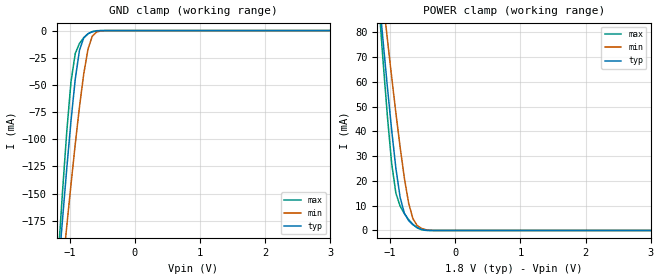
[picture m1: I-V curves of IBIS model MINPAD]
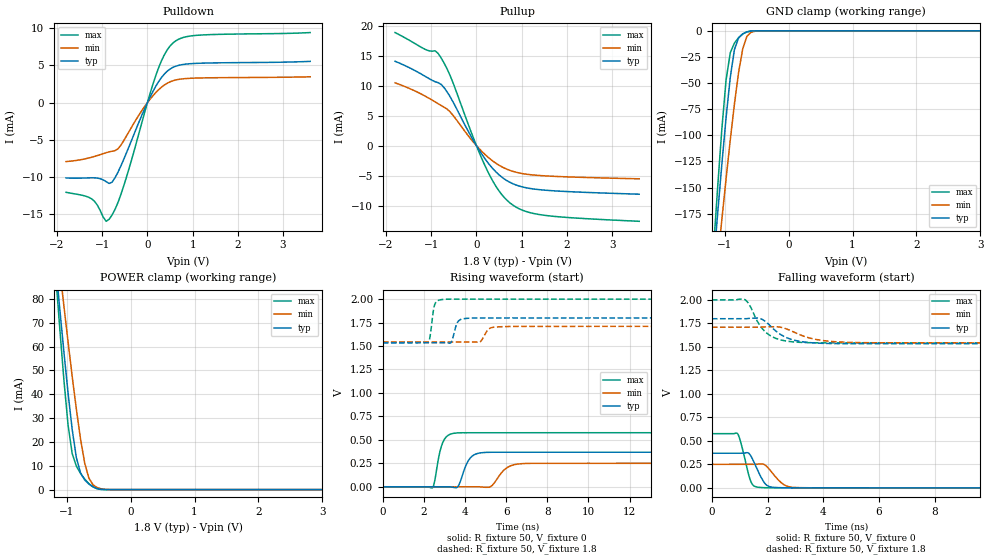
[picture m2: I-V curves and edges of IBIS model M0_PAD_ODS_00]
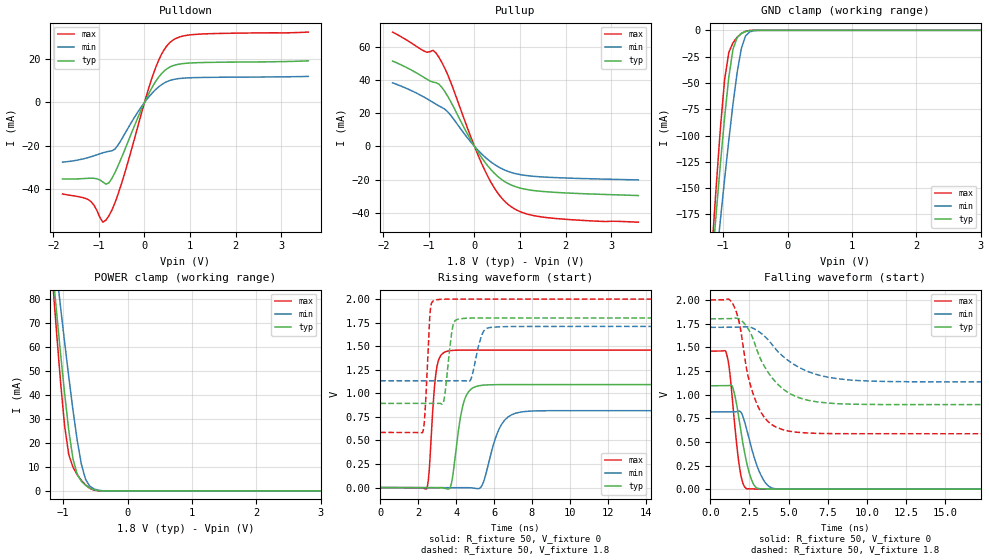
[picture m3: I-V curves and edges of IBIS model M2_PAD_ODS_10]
| Created by SiliconSmart  S-2021.06-SP5-2
[IBIS Ver]   4.0
[File Name]   as320ck_18v_rev1p1.ibs
[File Rev]   1.1
[Date]   Tue Aug 20 2024
|[Source]   Avalanche Team
|[Notes]   Generated IBIS models from Silicon Smart
|[Rev 1.0]   Initial release based on extracted netlist
|[Rev 1.1]   Updated the VCC supply values according to
|		datasheet
|[Disclaimer]   THE MODEL LIBRARIES ARE PROVIDED AS IS.
|[Copyright]   Copyright 2024, Avalanche Technology, All Rights Reserved
[Component]   AS30XX20X_BGA
[Manufacturer]  Avalanche Technology
| CONTENT :
| This file contains IBIS MODEL for PSRAM device
| AS30XX20X
| USAGE :
| The models are derived for the 1.71V to 2.0V I/O Operation.
| Temperatures for model generation: typ: 25, max: -40, min: 125
| Voltages : typ: 1.8V, min: 1.71V, max: 2.0V
| PACKAGES SUPPORTED :
| 56-ball FBGA (10mm x 10mm)
| VERIFICATION
| Errors  : 0
| Warnings: 11
| All warnings due to non-monotonic data:
[Package]
|  Design die-package: BGA
| variable   typ   min   max
R_pkg   0.72029   0.51528   1.0002
L_pkg   5.797e-9   4.155e-9   8.073e-9
C_pkg   1.116e-12   7.907e-13   1.753e-12
|Pin and Model info
[Pin]  signal_name  model_name   R_pin   L_pin   C_pin
E2   CS1#   MINPAD   0.4340	15.2000E-9	1.2600E-12
C3   CS2#   MINPAD   0.3800	13.5000E-9	1.0400E-12
D2   CLK1   MINPAD   0.4300	12.7000E-9	0.9790E-12
D1   CLK2   MINPAD   0.4480	14.6000E-9	1.1600E-12
F3   IO_0   MIOPAD   0.4010	12.4000E-9	1.2500E-12
F2   IO_1   MIOPAD   0.4050	14.2000E-9	1.1100E-12
E4   IO_2   MIOPAD   0.3780	11.8000E-9	1.2000E-12
F4   IO_3   MIOPAD   0.3700	11.8000E-9	1.2600E-12
F5   IO_4   MIOPAD   0.3710	11.1000E-9	1.1000E-12
G3   IO_5   MIOPAD   0.4050	13.8000E-9	1.1600E-12
G2   IO_6   MIOPAD   0.3830	15.2000E-9	1.0900E-12
G1   IO_7   MIOPAD   0.4480	16.4000E-9	1.0800E-12
C7   HTBSEL   MINPAD   0.1380	6.1700E-9	0.6060E-12
B7   HBP_2   MINPAD   0.1470	6.3900E-9	1.0000E-12
A6   HBP_1   MINPAD   0.1910	8.5000E-9	1.1500E-12
A5   HBP_0   MINPAD   0.2050	8.6800E-9	1.4200E-12
C4   RESET#   MINPAD   0.3410	14.1000E-9	1.6300E-12
C5   INT1#   MIOPAD   0.3080	12.5000E-9	1.2100E-12
D3   INT2#   MIOPAD   0.2120	10.3000E-9	0.8230E-12
B1   VSSIO   GND   NA   NA   NA
B5   VSSIO   GND   NA   NA   NA
B6   VSSIO   GND   NA   NA   NA
E1   VSSIO   GND   NA   NA   NA
G5   VSSIO   GND   NA   NA   NA
G6   VSSIO   GND   NA   NA   NA
A1   VSS   GND   NA   NA   NA
A3   VSS   GND   NA   NA   NA
B3   VSS   GND   NA   NA   NA
E5   VSS   GND   NA   NA   NA
E6   VSS   GND   NA   NA   NA
E7   VSS   GND   NA   NA   NA
G7   VSS   GND   NA   NA   NA
A8   VSS   GND   NA   NA   NA
A7   VCCIO   POWER   NA   NA   NA
B2   VCCIO   POWER   NA   NA   NA
B4   VCCIO   POWER   NA   NA   NA
C6   VCCIO   POWER   NA   NA   NA
F1   VCCIO   POWER   NA   NA   NA
F6   VCCIO   POWER   NA   NA   NA
G4   VCCIO   POWER   NA   NA   NA
A2   VCC   POWER   NA   NA   NA
A4   VCC   POWER   NA   NA   NA
D4   VCC   POWER   NA   NA   NA
D6   VCC   POWER   NA   NA   NA
D7   VCC   POWER   NA   NA   NA
F7   VCC   POWER   NA   NA   NA
| IOPAD
[Model Selector] MIOPAD
| Model Description
M0_PAD_ODS_00   35ohms
M1_PAD_ODS_01   40ohms
M2_PAD_ODS_10   20ohms
M3_PAD_ODS_11   15ohms
| Models and submodels in the file (5): MINPAD (Input), M0_PAD_ODS_00 (I/O), M2_PAD_ODS_10 (I/O), M1_PAD_ODS_01 (I/O), M3_PAD_ODS_11 (I/O)
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[Model] MINPAD
Model_type Input
Enable   Active-High
Vinl  =  0.63
Vinh  =  1.17
| Capacitance  typ   min   max
C_comp   1.623824e-12   1.523246e-12   1.739467e-12
| Variables   typ   min   max
[GND Clamp Reference]   0   0   0
[POWER Clamp Reference]   1.8   1.71   2
[Pulldown Reference]   0   0   0
[Pullup Reference]   1.8   1.71   2
[Temperature Range]   25   125   -40
[Voltage Range]   1.8   1.71   2
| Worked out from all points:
|   GND clamp passes 1 mA (typ) near -0.64 V on its own axis
|   POWER clamp passes 1 mA (typ) near -0.57 V on its own axis
[GND Clamp]
| Voltage   I(typ)   I(min)   I(max)
-1.8V     -720.4mA   -670.5mA   -825.2mA
-1.173V   -222.3mA   -260.3mA   -207.5mA
-1.108V   -173.8mA   -219.8mA   -148.3mA
-1.043V   -126.9mA   -180.1mA   -93.11mA
-977.6mV  -83.02mA   -141.5mA   -47mA
-912.4mV  -44.68mA   -104.6mA   -21.04mA
-847.2mV  -17.95mA   -70.1mA    -11.75mA
-782.1mV  -6.736mA   -39.85mA   -6.524mA
-716.9mV  -2.917mA   -17.13mA   -2.959mA
-651.7mV  -1.107mA   -5.246mA   -906.9uA
-456.2mV  -3.885uA   -74.14uA   -372.9nA
3.6V      0A         0A         0A
[POWER Clamp]
| Voltage   I(typ)   I(min)   I(max)
-1.8V     287.1mA    268.3mA    329.6mA
-1.173V   94.89mA    108.5mA    91.02mA
-1.108V   76.1mA     92.66mA    67.97mA
-1.043V   57.9mA     77.16mA    46.14mA
-977.6mV  40.62mA    62.05mA    27.14mA
-912.4mV  25.13mA    47.46mA    15.06mA
-847.2mV  13.38mA    33.64mA    9.853mA
-716.9mV  4.014mA    11.09mA    4.394mA
-651.7mV  2.34mA     4.821mA    2.483mA
-586.6mV  1.18mA     2.003mA    1.113mA
-325.9mV  1.153uA    19.85uA    110.1nA
3.6V      0A         0A         0A
[Model] M0_PAD_ODS_00
Model_type I/O
Enable   Active-High
Vinl  =  0.63
Vinh  =  1.17
Vmeas =  0.9
Cref  =  30e-12
| Capacitance  typ   min   max
C_comp   1.624629e-12   1.520611e-12   1.744819e-12
| Variables   typ   min   max
[GND Clamp Reference]   0   0   0
[POWER Clamp Reference]   1.8   1.71   2
[Pulldown Reference]   0   0   0
[Pullup Reference]   1.8   1.71   2
[Temperature Range]   25   125   -40
[Voltage Range]   1.8   1.71   2
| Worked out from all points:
|   slope of the pulldown table from 0 to 0.27 V, typ, clamps not added: 89.8 ohm
|   slope of the pullup table from 0 to 0.27 V, typ, clamps not added: 90.2 ohm
|   GND clamp passes 1 mA (typ) near -0.64 V on its own axis
|   POWER clamp passes 1 mA (typ) near -0.57 V on its own axis
|   falling waveform, R_fixture 50, V_fixture 0: 20-80 % time 364ps typ, 457ps min, 286ps max; typ from 0.368 V to 0 V
|   falling waveform, R_fixture 50, V_fixture 1.8: 20-80 % time 772ps typ, 993ps min, 609ps max; typ from 1.8 V to 1.53 V
|   rising waveform, R_fixture 50, V_fixture 0: 20-80 % time 416ps typ, 571ps min, 331ps max; typ from 0 V to 0.368 V
|   rising waveform, R_fixture 50, V_fixture 1.8: 20-80 % time 214ps typ, 282ps min, 164ps max; typ from 1.53 V to 1.8 V
[GND Clamp]
| Voltage   I(typ)   I(min)   I(max)
-1.8V     -720.4mA   -670.5mA   -825.2mA
-1.173V   -222.3mA   -260.3mA   -207.5mA
-1.108V   -173.8mA   -219.8mA   -148.3mA
-1.043V   -126.9mA   -180.1mA   -93.11mA
-977.6mV  -83.02mA   -141.5mA   -47.01mA
-912.4mV  -44.68mA   -104.6mA   -21.04mA
-847.2mV  -17.95mA   -70.1mA    -11.75mA
-782.1mV  -6.736mA   -39.85mA   -6.526mA
-716.9mV  -2.917mA   -17.13mA   -2.96mA
-651.7mV  -1.107mA   -5.246mA   -907.6uA
-456.2mV  -3.886uA   -74.14uA   -373.5nA
3.6V      0A         0A         0A
[POWER Clamp]
| Voltage   I(typ)   I(min)   I(max)
-1.8V     287.1mA    268.3mA    329.6mA
-1.173V   94.89mA    108.5mA    91.02mA
-1.108V   76.1mA     92.66mA    67.97mA
-1.043V   57.9mA     77.16mA    46.14mA
-977.6mV  40.62mA    62.05mA    27.14mA
-912.4mV  25.13mA    47.46mA    15.06mA
-847.2mV  13.38mA    33.64mA    9.853mA
-716.9mV  4.014mA    11.09mA    4.394mA
-651.7mV  2.34mA     4.821mA    2.483mA
-586.6mV  1.18mA     2.003mA    1.113mA
-325.9mV  1.153uA    19.85uA    110.1nA
3.6V      0A         0A         0A
[Pulldown]
| Voltage   I(typ)   I(min)   I(max)
-1.8V     -10.11mA   -7.903mA   -12.02mA
-1.238V   -10.08mA   -7.332mA   -12.89mA
-912.4mV  -10.6mA    -6.719mA   -15.91mA
-847.2mV  -10.84mA   -6.607mA   -15.64mA
-716.9mV  -10.08mA   -6.433mA   -14.32mA
-521.4mV  -7.576mA   -5.077mA   -11.12mA
-65.17mV  -872uA     -545.4uA   -1.404mA
248.3mV   2.817mA    1.73mA     4.683mA
434.5mV   4.193mA    2.586mA    7.041mA
620.7mV   4.869mA    3.026mA    8.258mA
1.179V    5.284mA    3.307mA    9.058mA
3.6V      5.531mA    3.462mA    9.391mA
[Pullup]
| Voltage   I(typ)   I(min)   I(max)
-1.8V     14.09mA    10.49mA    18.88mA
-1.108V   11.46mA    8.165mA    15.99mA
-912.4mV  10.68mA    7.305mA    15.83mA
-782.1mV  10.23mA    6.709mA    14.67mA
-586.6mV  8.225mA    5.675mA    11.78mA
-65.17mV  837.2uA    571.9uA    1.256mA
248.3mV   -2.788mA   -1.868mA   -4.273mA
496.6mV   -4.844mA   -3.246mA   -7.521mA
744.8mV   -6.13mA    -4.13mA    -9.572mA
1.055V    -6.951mA   -4.705mA   -10.87mA
1.49V     -7.407mA   -5.024mA   -11.6mA
3.6V      -8.097mA   -5.528mA   -12.62mA
[Ramp]
dV/dt_r   0.221023/0.415541n  0.150294/0.570736n  0.34588/0.331259n
dV/dt_f   0.159898/0.772458n  0.100157/0.992769n  0.274317/0.608956n
R_load = 50
[Falling Waveform]
R_fixture = 50
V_fixture = 0
V_fixture_min = 0
V_fixture_max = 0
| Time   V(typ)   V(min)   V(max)
0s        368.4mV    250.5mV    576.5mV
917.7ps   368.8mV    250.7mV    577.9mV
1.025ns   368.8mV    250.8mV    496.9mV
1.4ns     338.8mV    250.9mV    66.57mV
1.498ns   281.8mV    250.9mV    22.51mV
1.747ns   123.1mV    255.1mV    3.988mV
2.065ns   13.03mV    196.9mV    1.112mV
2.606ns   1.316mV    29.83mV    229.5uV
3.024ns   433.5uV    3.545mV    224.5uV
21.88ns   79.75nV    25.29nV    -226nV
[Falling Waveform]
R_fixture = 50
V_fixture = 1.8
V_fixture_min = 1.71
V_fixture_max = 2
| Time   V(typ)   V(min)   V(max)
0s        1.8V       1.71V      2V
1.175ns   1.8V       1.71V      2.005V
1.306ns   1.803V     1.71V      1.967V
1.72ns    1.803V     1.711V     1.731V
1.981ns   1.756V     1.714V     1.644V
2.418ns   1.642V     1.711V     1.579V
2.948ns   1.572V     1.658V     1.552V
3.916ns   1.539V     1.571V     1.544V
5.337ns   1.534V     1.546V     1.543V
21.88ns   1.534V     1.543V     1.543V
[Rising Waveform]
R_fixture = 50
V_fixture = 0
V_fixture_min = 0
V_fixture_max = 0
| Time   V(typ)   V(min)   V(max)
0s        2.923nV    85.23nV    2.501nV
2.41ns    -265.6uV   -270.7uV   -11.22mV
2.91ns    -320.8uV   -327uV     469.9mV
3.456ns   -7.235mV   -388.3uV   570.2mV
3.683ns   11.84mV    -413.8uV   574.5mV
4.261ns   309.1mV    -478.8uV   575.7mV
4.837ns   363.6mV    -3.076mV   575.7mV
6.059ns   367.9mV    206.6mV    575.8mV
6.73ns    367.9mV    245.7mV    575.8mV
21.88ns   368.4mV    250.5mV    576.5mV
[Rising Waveform]
R_fixture = 50
V_fixture = 1.8
V_fixture_min = 1.71
V_fixture_max = 2
| Time   V(typ)   V(min)   V(max)
0s        1.534V     1.543V     1.543V
2.209ns   1.534V     1.543V     1.54V
2.511ns   1.534V     1.543V     1.934V
2.877ns   1.534V     1.543V     1.996V
3.303ns   1.535V     1.543V     2V
3.663ns   1.763V     1.543V     2V
4.153ns   1.796V     1.542V     2V
4.701ns   1.799V     1.542V     2V
5.68ns    1.799V     1.705V     2V
21.88ns   1.8V       1.71V      2V
[Model] M2_PAD_ODS_10
Model_type I/O
Enable   Active-High
Vinl  =  0.63
Vinh  =  1.17
Vmeas =  0.9
Cref  =  30e-12
| Capacitance  typ   min   max
C_comp   1.624629e-12   1.520611e-12   1.744819e-12
| Variables   typ   min   max
[GND Clamp Reference]   0   0   0
[POWER Clamp Reference]   1.8   1.71   2
[Pulldown Reference]   0   0   0
[Pullup Reference]   1.8   1.71   2
[Temperature Range]   25   125   -40
[Voltage Range]   1.8   1.71   2
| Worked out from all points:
|   slope of the pulldown table from 0 to 0.27 V, typ, clamps not added: 25.7 ohm
|   slope of the pullup table from 0 to 0.27 V, typ, clamps not added: 24.7 ohm
|   GND clamp passes 1 mA (typ) near -0.64 V on its own axis
|   POWER clamp passes 1 mA (typ) near -0.57 V on its own axis
|   falling waveform, R_fixture 50, V_fixture 0: 20-80 % time 706ps typ, 900ps min, 524ps max; typ from 1.09 V to 0 V
|   falling waveform, R_fixture 50, V_fixture 1.8: 20-80 % time 1.87ns typ, 2.55ns min, 1.16ns max; typ from 1.8 V to 0.893 V
|   rising waveform, R_fixture 50, V_fixture 0: 20-80 % time 477ps typ, 754ps min, 290ps max; typ from 0 V to 1.09 V
|   rising waveform, R_fixture 50, V_fixture 1.8: 20-80 % time 292ps typ, 399ps min, 203ps max; typ from 0.893 V to 1.8 V
[GND Clamp]
| Voltage   I(typ)   I(min)   I(max)
-1.8V     -720.4mA   -670.5mA   -825.2mA
-1.173V   -222.3mA   -260.3mA   -207.5mA
-1.108V   -173.8mA   -219.8mA   -148.3mA
-1.043V   -126.9mA   -180.1mA   -93.11mA
-977.6mV  -83.02mA   -141.5mA   -47.01mA
-912.4mV  -44.68mA   -104.6mA   -21.04mA
-847.2mV  -17.95mA   -70.1mA    -11.75mA
-782.1mV  -6.736mA   -39.85mA   -6.526mA
-716.9mV  -2.917mA   -17.13mA   -2.96mA
-651.7mV  -1.107mA   -5.246mA   -907.6uA
-456.2mV  -3.886uA   -74.14uA   -373.5nA
3.6V      0A         0A         0A
[POWER Clamp]
| Voltage   I(typ)   I(min)   I(max)
-1.8V     287.1mA    268.3mA    329.6mA
-1.173V   94.89mA    108.5mA    91.02mA
-1.108V   76.1mA     92.66mA    67.97mA
-1.043V   57.9mA     77.16mA    46.14mA
-977.6mV  40.62mA    62.05mA    27.14mA
-912.4mV  25.13mA    47.46mA    15.06mA
-847.2mV  13.38mA    33.64mA    9.853mA
-716.9mV  4.014mA    11.09mA    4.394mA
-651.7mV  2.34mA     4.821mA    2.483mA
-586.6mV  1.18mA     2.003mA    1.113mA
-325.9mV  1.153uA    19.85uA    110.1nA
3.6V      0A         0A         0A
[Pulldown]
| Voltage   I(typ)   I(min)   I(max)
-1.8V     -35.5mA    -27.69mA   -42.5mA
-1.238V   -35.21mA   -25.6mA    -45.07mA
-912.4mV  -36.94mA   -23.37mA   -55.58mA
-847.2mV  -37.92mA   -22.98mA   -54.63mA
-716.9mV  -35.27mA   -22.46mA   -50mA
-521.4mV  -26.49mA   -17.75mA   -38.78mA
-65.17mV  -3.048mA   -1.907mA   -4.891mA
248.3mV   9.844mA    6.047mA    16.33mA
434.5mV   14.66mA    9.037mA    24.58mA
620.7mV   17.01mA    10.57mA    28.86mA
1.179V    18.47mA    11.56mA    31.67mA
3.6V      19.32mA    12.09mA    32.66mA
[Pullup]
| Voltage   I(typ)   I(min)   I(max)
-1.8V     51.33mA    38.22mA    68.75mA
-1.108V   41.45mA    29.65mA    57.3mA
-912.4mV  38.66mA    26.5mA     57.78mA
-782.1mV  37.42mA    24.38mA    53.62mA
-586.6mV  30.08mA    20.75mA    43.03mA
-65.17mV  3.06mA     2.09mA     4.59mA
248.3mV   -10.19mA   -6.826mA   -15.61mA
496.6mV   -17.7mA    -11.86mA   -27.5mA
744.8mV   -22.4mA    -15.09mA   -35.02mA
1.055V    -25.41mA   -17.19mA   -39.79mA
1.49V     -27.08mA   -18.35mA   -42.46mA
3.6V      -29.55mA   -20.16mA   -45.58mA
[Ramp]
dV/dt_r   0.655597/0.476918n  0.489635/0.75417n  0.875432/0.290065n
dV/dt_f   0.544074/1.87057n  0.346028/2.55295n  0.848876/1.15854n
R_load = 50
[Falling Waveform]
R_fixture = 50
V_fixture = 0
V_fixture_min = 0
V_fixture_max = 0
| Time   V(typ)   V(min)   V(max)
0s        1.093V     816.1mV    1.459V
1.052ns   1.093V     816.2mV    1.422V
1.251ns   1.097V     816.2mV    1.226V
1.438ns   1.072V     816.3mV    896.6mV
1.876ns   696.7mV    823.6mV    218.5mV
2.331ns   273.5mV    626.7mV    4.167mV
2.894ns   21.69mV    287.4mV    1.151mV
3.495ns   1.982mV    72.91mV    837.6uV
4.044ns   895.6uV    7.213mV    812.3uV
21.88ns   -2.321uV   906.9nV    -6.953uV
[Falling Waveform]
R_fixture = 50
V_fixture = 1.8
V_fixture_min = 1.71
V_fixture_max = 2
| Time   V(typ)   V(min)   V(max)
0s        1.8V       1.71V      2V
1.454ns   1.806V     1.711V     1.955V
1.823ns   1.8V       1.711V     1.78V
2.37ns    1.708V     1.716V     1.224V
2.755ns   1.577V     1.698V     995.7mV
3.431ns   1.304V     1.621V     762.3mV
4.221ns   1.124V     1.471V     653mV
5.692ns   964.8mV    1.284V     599.3mV
8.117ns   903.2mV    1.167V     586.4mV
21.88ns   893.2mV    1.133V     585.2mV
[Rising Waveform]
R_fixture = 50
V_fixture = 0
V_fixture_min = 0
V_fixture_max = 0
| Time   V(typ)   V(min)   V(max)
0s        1.933nV    49.93nV    1.563nV
2.448ns   -325uV     -312.3uV   -10.12mV
2.965ns   -393.6uV   -378.3uV   1.255V
3.533ns   -13.78mV   -450.7uV   1.447V
3.784ns   76.06mV    -482.7uV   1.455V
4.401ns   904.4mV    -561.5uV   1.459V
5.009ns   1.07V      -9.749mV   1.459V
6.326ns   1.092V     645.2mV    1.459V
7.129ns   1.093V     788.3mV    1.459V
21.88ns   1.093V     816.1mV    1.459V
[Rising Waveform]
R_fixture = 50
V_fixture = 1.8
V_fixture_min = 1.71
V_fixture_max = 2
| Time   V(typ)   V(min)   V(max)
0s        893.2mV    1.133V     585.2mV
2.244ns   893.9mV    1.134V     590.6mV
2.636ns   894mV      1.134V     1.876V
2.902ns   894.1mV    1.134V     1.989V
3.336ns   908mV      1.134V     1.999V
3.785ns   1.668V     1.134V     2V
4.117ns   1.787V     1.134V     2V
4.758ns   1.798V     1.14V      2V
5.739ns   1.799V     1.697V     2V
21.88ns   1.8V       1.71V      2V
